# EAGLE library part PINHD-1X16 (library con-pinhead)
PIN HEADER
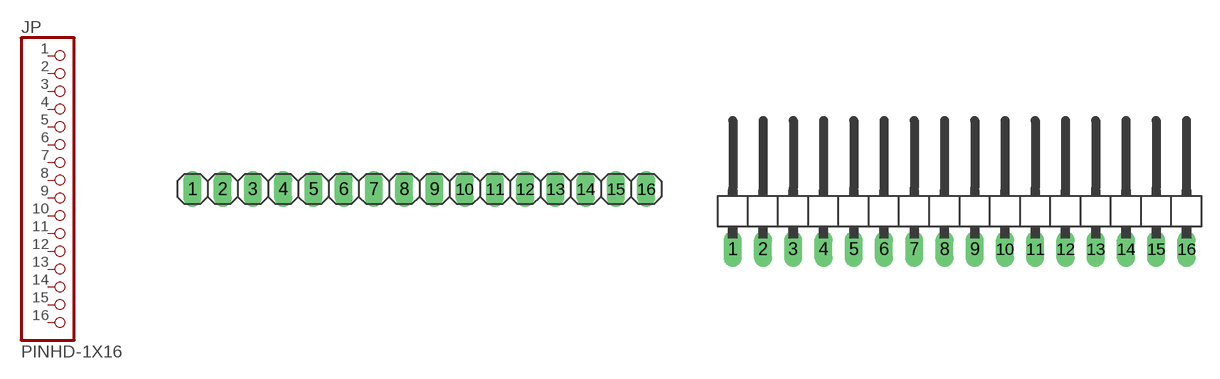
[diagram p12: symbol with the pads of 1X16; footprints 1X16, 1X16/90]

Designator prefix JP

## PINHD-1X16_2.54  [1X16]
1  1  pas
2  2  pas
3  3  pas
4  4  pas
5  5  pas
6  6  pas
7  7  pas
8  8  pas
9  9  pas
10  10  pas
11  11  pas
12  12  pas
13  13  pas
14  14  pas
15  15  pas
16  16  pas

## PINHD-1X16_2.54-90°  [1X16/90]
Pads as for 1X16

## PINHD-1X16_2.00  [1X16M]
Pads as for 1X16

## PINHD-1X16_2.54-SMD  [1X16SMD]
Pads as for 1X16

## PINHD-1X16_2.54-SMD-90°  [1X16SMD/90]
Pads as for 1X16

## Footprint 1X16 (pad centres in mm)
PIN HEADER - 2.54
drill 1.016 long: 1 -19.05,0; 2 -16.51,0; 3 -13.97,0; 4 -11.43,0; 5 -8.89,0; 6 -6.35,0; 7 -3.81,0; 8 -1.27,0; 9 1.27,0; 10 3.81,0; 11 6.35,0; 12 8.89,0; 13 11.43,0; 14 13.97,0; 15 16.51,0; 16 19.05,0

## Footprint 1X16/90 (pad centres in mm)
PIN HEADER - 2.54 90°
drill 1.016 long: 1 -19.05,-3.81; 2 -16.51,-3.81; 3 -13.97,-3.81; 4 -11.43,-3.81; 5 -8.89,-3.81; 6 -6.35,-3.81; 7 -3.81,-3.81; 8 -1.27,-3.81; 9 1.27,-3.81; 10 3.81,-3.81; 11 6.35,-3.81; 12 8.89,-3.81; 13 11.43,-3.81; 14 13.97,-3.81; 15 16.51,-3.81; 16 19.05,-3.81

## Footprint 1X16M (pad centres in mm)
PIN HEADER - 2
drill 0.914 square: 1 -15,0
drill 0.914: 2 -13,0; 3 -11,0; 4 -9,0; 5 -7,0; 6 -5,0; 7 -3,0; 8 -1,0; 9 1,0; 10 3,0; 11 5,0; 12 7,0; 13 9,0; 14 11,0; 15 13,0; 16 15,0

## Footprint 1X16SMD (pad centres in mm)
PIN HEADER - 2.54 SMD
smd 1.016 x 3.302: 1 -1.27,1.27; 2 1.27,-1.27; 3 3.81,1.27; 4 6.35,-1.27; 5 8.89,1.27; 6 11.43,-1.27; 7 13.97,1.27; 8 16.51,-1.27; 9 19.05,1.27; 10 21.59,-1.27; 11 24.13,1.27; 12 26.67,-1.27; 13 29.21,1.27; 14 31.75,-1.27; 15 34.29,1.27; 16 36.83,-1.27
